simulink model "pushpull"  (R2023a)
settings: Solver=VariableStepAuto  StartTime=0.0  StopTime=0.1  RelTol=1e-3
libraries: spsDiodeLib x4, spsMosfetLib x2, spsSeriesRLCBranchLib x2, spsDCVoltageSourceLib x1, spsGroundLib x1, spsLinearTransformerLib x1, spsVoltageMeasurementLib x1, sps_lib x1

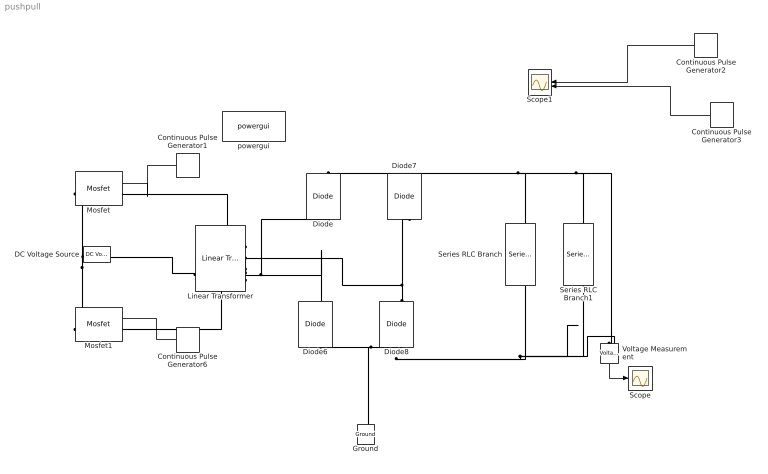
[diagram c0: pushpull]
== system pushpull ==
  Continuous Pulse Generator1 : DiscretePulseGenerator  PulseType=Time based  Period=35.714e-6  PulseWidth=45
  Continuous Pulse Generator2 : DiscretePulseGenerator  PulseType=Time based  Period=35.714e-6  PulseWidth=45
  Continuous Pulse Generator3 : DiscretePulseGenerator  PulseType=Time based  Period=35.714e-6  PulseWidth=45  PhaseDelay=17.857e-6
  Continuous Pulse Generator6 : DiscretePulseGenerator  PulseType=Time based  Period=35.714e-6  PulseWidth=45  PhaseDelay=17.857e-6
  DC Voltage Source : spsDCVoltageSourceLib/DC Voltage Source  Amplitude=12  Measurements=None
  Diode{,6..8} (4 alike) : spsDiodeLib/Diode  Ron=0.001  Lon=0  Vf=0.8  IC=0  UseSnubber=0  Rs=500  Cs=250e-9  Measurements=on
  Ground : spsGroundLib/Ground  LConnTagsString=a
  Linear Transformer : spsLinearTransformerLib/Linear Transformer  UNITS=SI  NominalPower=[ 250e6 60 ]  winding1=[31 0 0]  winding2=[1 0 0]  ThreeWindings=on  winding3=[1 0 0]  RmLm=[inf inf]  Measurements=None  DataType=on
  Mosfet : spsMosfetLib/Mosfet  Ron=0.1  Lon=0  Rd=0.01  Vfd=0  IC=0  Rs=1e5  Cs=inf  Measurements=on
  Mosfet1 : spsMosfetLib/Mosfet  Ron=0.1  Lon=0  Rd=0.01  Vfd=0  IC=0  Rs=1e5  Cs=inf  Measurements=on
  Scope : Scope
  Scope1 : Scope  NumInputPorts=2
  Series RLC Branch : spsSeriesRLCBranchLib/Series RLC Branch  LConnTagsString=__new0  RConnTagsString=__new0  BranchType=C  Resistance=1  Inductance=1e-3  SetiL0=off  InitialCurrent=0  Capacitance=0.47e-6  Setx0=off  InitialVoltage=0  Measurements=None
  Series RLC Branch1 : spsSeriesRLCBranchLib/Series RLC Branch  LConnTagsString=__new0  RConnTagsString=__new0  BranchType=R  Resistance=96.1  Inductance=1e-3  SetiL0=off  InitialCurrent=0  Capacitance=1e-6  Setx0=off  InitialVoltage=0  Measurements=None
  Voltage Measurement : spsVoltageMeasurementLib/Voltage Measurement  PhasorSimulation=off  OutputType=Complex  PSBequivalent=0
  powergui : sps_lib/powergui  Priority=1  SimulationMode=Continuous  SampleTime=50e-6  frequency=60  Iterations=50  frequencyindice=0  Pbase=100e6  ErrMax=1e-4  UnitsV=kV  UnitsW=MW  buscounter=0  FunctionMessages=off  echomessages=off  EnableUseOfTLC=off  CurrentSourceSwitches=off  DisableSnubberDevices=off  DisableRonSwitches=off  DisableVfSwitches=off  DisplayEquations=off  AutomaticDiscreteSolvers=off  SolverType=Tustin/Backward Euler (TBE)  Interpol=off  ExternalGateDelay=off  methode=off  Ts=100  x0status=blocks  SPID=on  SwTol=0  HookPort=off  NonlinearTolerance=1e-4  nMaxIteration=100  ContinueOnMaxIteration=off  RestoreLinks=warning  ResistiveCurrentMeasurement=off  Frange=[0:2:500]  Ylog=off  Xlog=on  ShowGrid=off  save=off  variable=ZData  structure=0  ZoomFFT=off  StartTime=0.0  cycles=1  DisplayStyle=1  fundamental=60  FreqAxis=off  MaxFrequency=1000  frequencyindicesteady=1  RmsSteady=1  display=off
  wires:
  Voltage Measurement/1 -> Scope/1
  Continuous Pulse Generator2/1 -> Scope1/1
  Continuous Pulse Generator3/1 -> Scope1/2
  Continuous Pulse Generator1/1 -> Mosfet/1
  Continuous Pulse Generator6/1 -> Mosfet1/1
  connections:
  Linear Transformer/RConn1 -- Mosfet1/LConn1
  Mosfet/RConn1 -- Mosfet1/RConn1 -- DC Voltage Source/LConn1
  Linear Transformer/RConn4 -- Mosfet/LConn1
  Linear Transformer/RConn3 -- Linear Transformer/RConn2 -- DC Voltage Source/RConn1
  Linear Transformer/LConn2 -- Diode/LConn1 -- Diode6/RConn1
  Diode6/LConn1 -- Ground/LConn1 -- Series RLC Branch1/RConn1 -- Voltage Measurement/LConn2 -- Series RLC Branch/RConn1 -- Diode8/LConn1
  Diode8/RConn1 -- Diode7/LConn1 -- Linear Transformer/LConn1
  Diode/RConn1 -- Series RLC Branch/LConn1 -- Series RLC Branch1/LConn1 -- Voltage Measurement/LConn1 -- Diode7/RConn1
